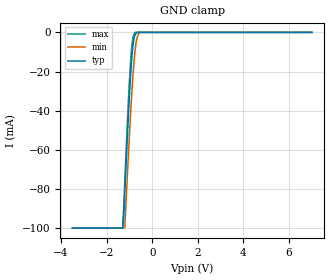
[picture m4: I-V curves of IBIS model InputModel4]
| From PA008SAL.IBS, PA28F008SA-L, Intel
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|**********************Input Model 4***************************************
[Model]   InputModel4
Model_type   Input
|   For RP#
Vinl = 0.8V
Vinh = 2.0V
| Variable   typ   min   max
C_comp   5.61p   NA   7.6p
[Voltage Range]   3.3V   3.0V   3.6V
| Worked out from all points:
|   GND clamp passes 1 mA (typ) near -0.74 V on its own axis
[GND_clamp]
|Voltage I(typ)   I(min)   I(max)
-3.5V     -100mA     -100mA     -100mA
-1.3V     -100mA     -100mA     -99.86mA
-1.25V    -94.3mA    -100mA     -89.26mA
-1.2V     -81.11mA   -99.61mA   -75.16mA
-1.05V    -43.96mA   -63.7mA    -36.21mA
-950mV    -22.5mA    -41.7mA    -14.95mA
-900mV    -13.72mA   -31.75mA   -7.337mA
-850mV    -7.248mA   -22.87mA   -2.883mA
-750mV    -1.125mA   -8.916mA   0A
-650mV    0A         -2.185mA   0A
-550mV    0A         0A         0A
7V        0A         0A         0A
[POWER_clamp]
| Input buffer circuits of this product do not intrinsically
| require a [POWER_clamp] definition.  This zero current
| [POWER_clamp] is provided for compatibility with some ibis
| parsers.
|Voltage  I(typ)   I(min)   I(max)
-3.3V     0A         0A         0A
0V        0A         0A         0A
3.3V      0A         0A         0A
6.6V      0A         0A         0A
